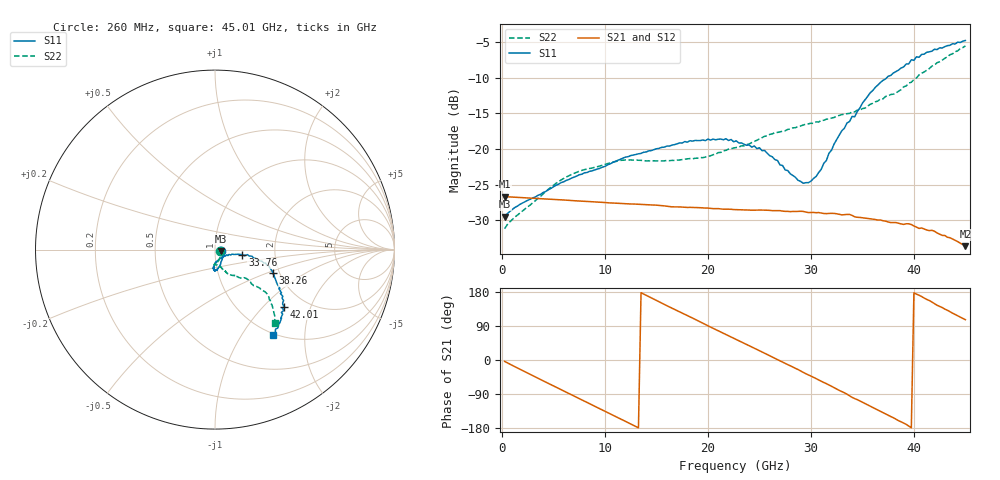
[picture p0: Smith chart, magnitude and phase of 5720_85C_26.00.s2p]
! Device:  ADRF5720
! Description: 0.5dB LSB GaAs MMIC 6-bit Digital Attenuator
! Frequency:  0.000009 -  40 GHz
! Ports:
!	RF1	= Port 1
!	RF2	= Port 2
! Vdd:  3.3 Volt
! Vss:  -3.3 Volt
! Control:  0/3.3 Volt
! State:  26.00 dB attenuation
! Data:  The device was measured using G-S-G Probes on a matrix board.
!  Data was collected using an calibrated 4 port network analyzer.
!  The reference plane for this measurement is at the launchers.
! Note:  Analog Devices supplies this data as a sample of measured data
!  for this product.  Your particular data for this product may vary.
!  Data was taken at 85 degrees C.
!  Analog Devices reserves the right to change this data at anytime.
# GHZ S DB R 45.0
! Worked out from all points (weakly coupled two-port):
!   180 points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, 260 MHz to 45.01 GHz, reference 45 ohm
!   highest |S21| = -26.68 dB at 260 MHz (marker M1); lowest = -33.6 dB at 45.01 GHz (marker M2)
!   lowest |S11| = -29.5 dB at 260 MHz (marker M3), VSWR 1.07, Z = 48 - j0.786 ohm
!   |S11| at or under -10 dB: start of sweep to 37.39 GHz
!   |S22| runs from -31.2 to -5.6 dB; largest |S21 - S12| = 0.00028
!   S11 on the Smith chart (normalised r, x): 260 MHz: 1.07, -0.02; 33.76 GHz: 1.36, -0.09; 38.26 GHz: 1.84, -0.55; 42.01 GHz: 1.57, -1.33; 45.01 GHz: 0.97, -1.39
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0.26  -29.51 -14.2  -26.68 -3.8  -26.68 -3.8  -31.18 -17.8
1.26  -28.20 -3.8  -26.77 -17.7  -26.76 -17.7  -29.55 -12.0
5.01  -25.30 -37.6  -27.08 -68.4  -27.06 -68.4  -25.08 -61.9
7.76  -23.55 -52.7  -27.32 -105.3  -27.30 -105.2  -23.01 -78.2
11.51  -21.44 -68.3  -27.64 -155.4  -27.63 -155.3  -21.61 -91.6
15.26  -19.92 -77.9  -27.92 153.7  -27.91 153.8  -21.67 -92.8
18.26  -18.85 -84.5  -28.19 114.0  -28.18 114.1  -21.35 -86.5
22.76  -18.86 -92.2  -28.51 54.0  -28.49 54.2  -19.81 -72.8
25.51  -20.22 -93.0  -28.58 17.8  -28.56 18.1  -18.23 -68.4
29.26  -24.81 -59.6  -28.76 -32.6  -28.75 -32.3  -16.65 -63.0
30.26  -24.14 -40.8  -28.90 -45.7  -28.88 -45.4  -16.43 -61.9
31.01  -22.85 -23.8  -28.99 -56.1  -28.97 -55.8  -16.00 -60.5
33.01  -17.45 -11.2  -29.25 -83.4  -29.23 -83.1  -15.19 -56.1
33.76  -16.16 -11.3  -29.18 -94.5  -29.17 -94.2  -15.02 -53.5
34.26  -15.49 -12.0  -29.52 -101.9  -29.49 -101.7  -14.81 -52.4
35.76  -12.15 -13.2  -29.81 -121.6  -29.77 -121.3  -13.75 -49.5
37.76  -9.70 -19.0  -30.32 -149.2  -30.29 -148.8  -12.37 -42.9
38.26  -9.17 -22.4  -30.32 -156.2  -30.30 -155.8  -12.18 -42.3
40.26  -7.09 -33.0  -30.96 173.7  -30.94 174.0  -10.06 -41.3
42.01  -6.03 -39.5  -31.54 148.5  -31.52 149.0  -8.24 -40.8
43.51  -5.48 -45.8  -32.45 127.5  -32.42 128.0  -6.80 -45.3
45.01  -4.80 -56.1  -33.63 106.3  -33.55 106.8  -5.57 -50.6
